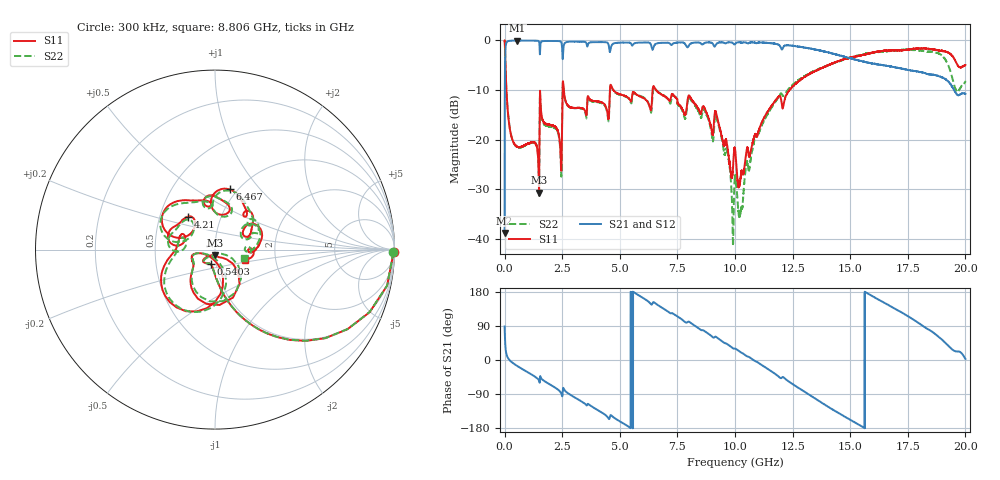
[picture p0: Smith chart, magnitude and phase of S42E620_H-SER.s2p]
! Created Wed Nov 25 22:22:17 2020
# khz S ma R 50
! 2 Port Network Data from SP1.SP block
! freq  magS11  angS11  magS21  angS21  magS12  angS12  magS22  angS22
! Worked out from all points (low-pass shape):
!   20001 points, 300 kHz to 20 GHz, reference 50 ohm
!   highest |S21| = -0.04 dB at 553.3 MHz (marker M1); lowest = -38.8 dB at 300 kHz (marker M2)
!   |S21| within 3 dB of the highest: 26.01 MHz to 2.51 GHz (2.484 GHz wide, 196 % of centre); 2.534 GHz to 14.53 GHz (12 GHz wide, 141 % of centre)
!   lowest |S11| = -30.7 dB at 1.495 GHz (marker M3), VSWR 1.06, Z = 50 - j2.93 ohm
!   |S11| at or under -10 dB: 79.12 MHz to 2.514 GHz (2.434 GHz wide, 188 % of centre); 2.57 GHz to 4.57 GHz (2 GHz wide, 56 % of centre); 6.576 GHz to 12.36 GHz (5.789 GHz wide, 61.1 % of centre)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
!   |S22| runs from -41.4 to 0.0 dB; largest |S21 - S12| = 0.018
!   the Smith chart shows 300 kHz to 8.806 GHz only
!   S11 on the Smith chart (normalised r, x): 300 kHz: open; 540.3 MHz: 0.94, -0.15; 4.21 GHz: 0.69, +0.27; 6.467 GHz: 0.92, +0.70; 8.806 GHz: 1.39, -0.16
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300  0.9959 -0.7  0.01149 88.4  0.01141 89.5  0.9941 -0.8
112300  0.2321 -80.9  0.9718 9.2  0.9722 9.2  0.233 -80.8
540300  0.0849 -106.4  0.9953 -15.4  0.9953 -15.5  0.08466 -105.9
553300  0.08477 -106.8  0.9958 -15.9  0.995 -15.9  0.08422 -106.3
1495300  0.02925 -88.2  0.9699 -54.8  0.9699 -54.8  0.02977 -85.5
1618300  0.1681 -138.2  0.9775 -50.5  0.978 -50.5  0.1618 -139.7
2392300  0.09753 -168.1  0.9811 -82.3  0.982 -82.3  0.09388 -168.1
2601300  0.2746 -166.8  0.9325 -79.3  0.9325 -79.3  0.2709 -162.3
3334300  0.2082 157.7  0.9706 -109.2  0.9707 -109.2  0.2067 164.3
4210300  0.238 129.5  0.962 -138.3  0.9617 -138.2  0.2336 135.3
6467300  0.3453 76.3  0.8611 152.8  0.8589 152.7  0.3389 75.2
6667300  0.3002 58.5  0.939 144.3  0.9362 144.2  0.3021 54.1
8806300  0.1764 -18.2  0.9546 71.1  0.9551 70.9  0.1694 -15.9
1.00003e7  0.08138 -3.6  0.9171 30.2  0.9173 30.3  0.04265 -21.4
1.02483e7  0.04201 41.4  0.9527 20.2  0.9536 20.2  0.01933 156.5
1.13583e7  0.182 61.0  0.9434 -21.1  0.9429 -21.2  0.1709 69.5
1.33343e7  0.4723 -4.4  0.822 -96.1  0.8254 -96.0  0.4781 -8.9
1.48023e7  0.6486 -60.1  0.68 -150.7  0.6794 -151.1  0.6492 -62.6
1.66673e7  0.7884 -120.9  0.5533 144.9  0.5402 145.1  0.7818 -128.3
1.80683e7  0.8253 -172.1  0.4799 93.5  0.4824 94.6  0.7922 -176.0
1.90943e7  0.7767 147.5  0.4112 47.5  0.4118 47.3  0.6587 139.9
2e7  0.566 140.5  0.2881 2.8  0.2867 3.1  0.3853 155.5
